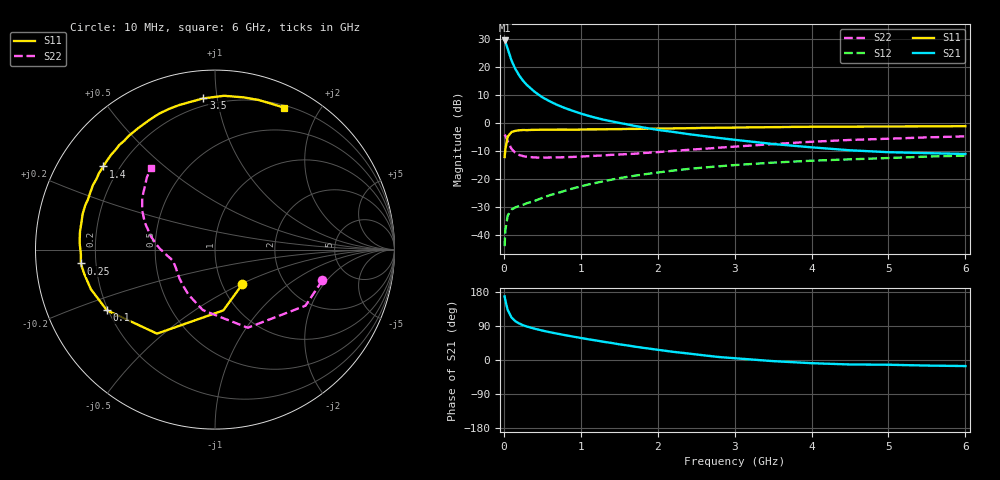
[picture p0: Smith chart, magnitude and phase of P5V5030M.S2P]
! SIEMENS Small Signal Semiconductors
! BFP183
! Si NPN RF Bipolar Junction Transistor in SOT143
! VCE = 0.5 V  IC = 30 mA
! Common Emitter S-Parameters:  March  1996
# GHz  S  MA  R  50
!  f  S11  S21  S12  S22
! GHz  MAG  ANG  MAG  ANG  MAG  ANG  MAG  ANG
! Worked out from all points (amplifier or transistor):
!   36 points, 10 MHz to 6 GHz, reference 50 ohm
!   highest |S21| = 29.6 dB at 10 MHz (marker M1)
!   |S21| within 3 dB of that: start of sweep to 49.79 MHz
!   unconditionally stable (mu >= 1): start of sweep to 16.33 MHz; 214.2 MHz to end of sweep
!   at 250 MHz: K = 1.11, MAG = 20.3 dB, |S12| = -29.3 dB
!   at 1.4 GHz: K = 1.95, MAG = 4.9 dB, |S12| = -20.3 dB
!   at 6 GHz: K = 1.53, MAG = -4.0 dB, |S12| = -11.7 dB
!   S11 on the Smith chart (normalised r, x): 10 MHz: 1.25, -0.51; 100 MHz: 0.19, -0.25; 250 MHz: 0.14, -0.05; 1.4 GHz: 0.14, +0.33; 3.5 GHz: 0.16, +0.91; 6 GHz: 0.23, +1.58
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0.01  0.2457 -51.5  30.27 167.9  0.0062 72.8  0.6225 -16.0
0.02  0.3419 -82.2  28.67 156.9  0.0121 65.0  0.593 -31.8
0.05  0.5688 -124.6  21.39 132.0  0.0219 48.9  0.472 -67.3
0.1  0.691 -150.7  13.18 112.1  0.0281 35.9  0.344 -101.3
0.15  0.7258 -162.3  9.317 102.3  0.0308 33.2  0.2915 -120.4
0.2  0.7403 -169.2  7.108 96.3  0.0327 34.2  0.2677 -132.1
0.25  0.7517 -174.1  5.733 91.8  0.0342 35.3  0.2555 -140.3
0.3  0.7476 -177.8  4.812 88.3  0.0365 38.1  0.2483 -146.1
0.4  0.7556 176.9  3.639 82.6  0.0403 41.4  0.2416 -153.1
0.5  0.759 172.2  2.898 77.7  0.0455 44.4  0.2401 -157.8
0.6  0.7594 168.4  2.44 73.3  0.051 47.0  0.2413 -161.1
0.7  0.7637 164.9  2.095 69.3  0.0556 49.0  0.2425 -163.5
0.9  0.761 158.4  1.65 61.8  0.0675 50.8  0.2469 -166.4
1.1  0.7692 152.0  1.347 54.6  0.0793 51.3  0.2549 -169.4
1.4  0.7756 143.3  1.074 45.0  0.0966 50.1  0.2693 -172.9
1.8  0.7899 132.5  0.84 32.5  0.1191 47.0  0.2894 -177.2
2.2  0.8007 122.3  0.694 21.6  0.1404 42.5  0.3162 177.2
2.8  0.8247 108.1  0.54 7.8  0.1679 35.3  0.3624 168.8
3.5  0.845 94.4  0.421 -3.0  0.1954 27.2  0.4203 158.7
4.5  0.8629 79.4  0.325 -11.8  0.2235 16.0  0.498 144.5
5.5  0.8714 68.7  0.289 -14.7  0.2506 6.6  0.5533 133.3
6  0.8798 64.0  0.279 -16.0  0.2604 1.5  0.5774 128.1
